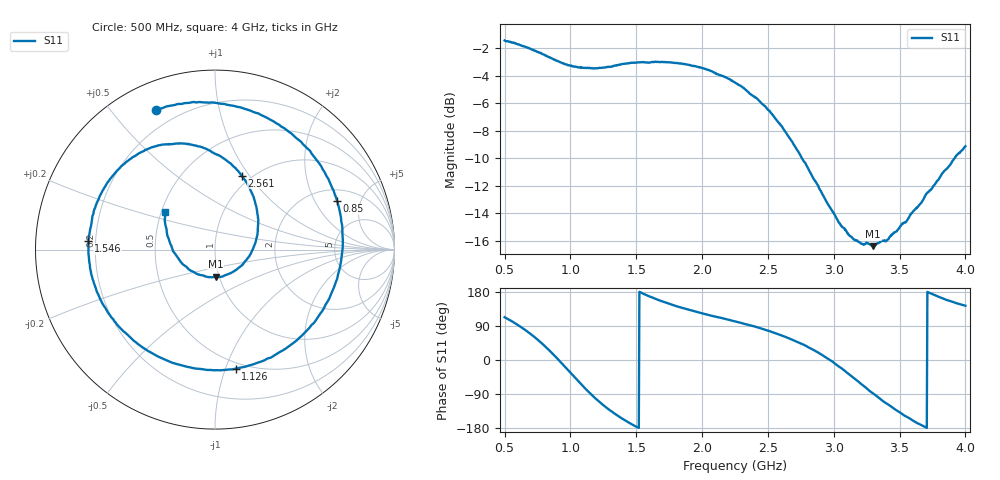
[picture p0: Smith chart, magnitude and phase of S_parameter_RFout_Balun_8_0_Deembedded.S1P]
!Agilent Technologies,E5071B,MY42403504,A.06.51
!Date: Wed Feb 26 14:56:26 2014
!Data & Calibration Information:
!Freq	S11:SOLT1(ON)
# Hz S dB R 50
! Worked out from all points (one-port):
!   801 points, 500 MHz to 4 GHz, reference 50 ohm
!   lowest |S11| = -16.4 dB at 3.3 GHz (marker M1), VSWR 1.36, Z = 48.1 - j14.9 ohm
!   |S11| at or under -10 dB: 2.758 GHz to 3.918 GHz (1.16 GHz wide, 34.7 % of centre)
!   S11 on the Smith chart (normalised r, x): 500 MHz: 0.12, +0.66; 850 MHz: 2.65, +3.09; 1.126 GHz: 0.45, -1.09; 1.546 GHz: 0.17, +0.03; 2.561 GHz: 0.90, +0.92; 4 GHz: 0.52, +0.25
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5e8  -1.44 112.9
6.00625e8  -1.73 92.4
6.8375e8  -1.98 72.3
7.625e8  -2.33 50.2
8.5e8  -2.71 21.6
8.9375e8  -2.92 6.3
9.375e8  -3.08 -9.8
9.85625e8  -3.23 -28.1
1.038125e9  -3.34 -48.1
1.125625e9  -3.44 -80.0
1.230625e9  -3.44 -113.7
1.29625e9  -3.35 -131.9
1.375e9  -3.20 -150.6
1.458125e9  -3.07 -168.0
1.545625e9  -3.02 176.1
1.676875e9  -3.01 157.3
1.8125e9  -3.08 141.2
2.0225e9  -3.51 121.2
2.25e9  -4.51 101.8
2.420625e9  -5.69 86.3
2.560625e9  -7.17 70.2
2.6875e9  -8.85 53.0
2.893125e9  -12.24 17.2
3.125e9  -15.66 -40.0
3.3e9  -16.39 -88.6
3.5625e9  -14.44 -151.4
3.7725e9  -11.83 170.5
4e9  -9.13 143.3
